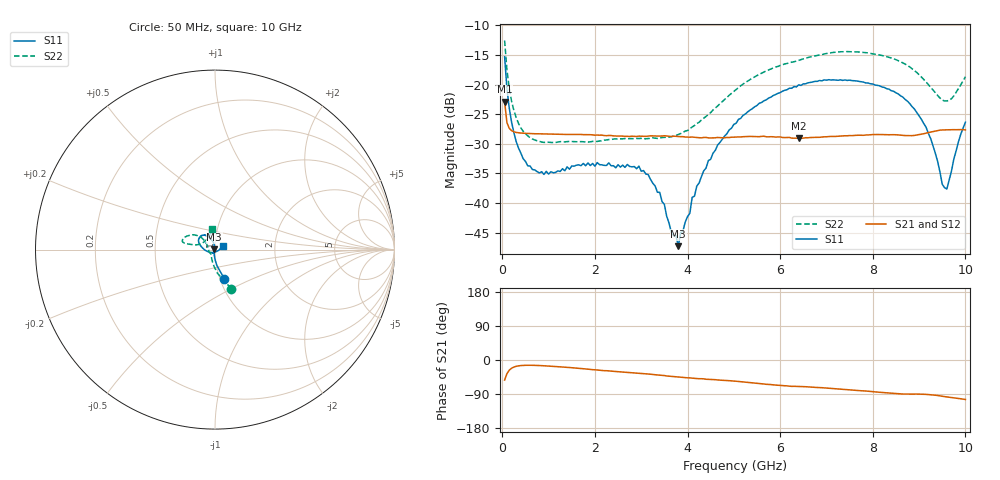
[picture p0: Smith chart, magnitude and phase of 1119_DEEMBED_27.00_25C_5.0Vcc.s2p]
!Hittite Microwave Corp.
!Digital Attenuator/PhaseShifter Rev 1.4.0
!Filename: C:\DATA\DATA\1119_DEEMBED_27.00_25C_5.0Vcc.s2p
!VNA ID: Agilent Technologies,N5224A,MY51441122,A.10.45.03
!Device type:
!2 Port Calibration.
!Temp(C): 25
!Lot Number:
!Serial Number:
!Operator:
!Misc:
!Attenuator:  27.000
# GHZ S DB R 50.0
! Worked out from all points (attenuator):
!   200 points, 50 MHz to 10 GHz, reference 50 ohm
!   highest |S21| = -22.89 dB at 50 MHz (marker M1); lowest = -29.1 dB at 6.4 GHz (marker M2)
!   lowest |S11| = -47.3 dB at 3.8 GHz (marker M3), VSWR 1.01, Z = 49.6 + j0.0687 ohm
!   |S11| at or under -10 dB: start of sweep to end of sweep
!   |S22| runs from -29.8 to -12.6 dB; largest |S21 - S12| = 0.00013
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0.05  -15.31 -72.2  -22.89 -53.0  -22.90 -53.0  -12.56 -67.4
0.1  -20.72 -82.6  -26.42 -36.2  -26.41 -36.1  -17.51 -83.9
0.2  -26.33 -91.3  -27.78 -21.7  -27.78 -21.7  -22.79 -100.5
0.35  -30.72 -98.1  -28.14 -15.5  -28.15 -15.5  -26.56 -114.7
0.55  -33.72 -106.2  -28.26 -13.8  -28.26 -13.9  -28.66 -126.3
0.9  -35.18 -113.4  -28.34 -15.2  -28.35 -15.2  -29.77 -135.8
1.75  -33.32 -121.9  -28.46 -23.1  -28.46 -23.1  -29.66 -140.7
2.95  -33.78 -113.3  -28.71 -34.8  -28.72 -34.9  -29.12 -160.0
3.4  -38.20 -124.2  -28.69 -39.8  -28.70 -39.9  -29.02 -173.5
3.8  -47.29 170.8  -28.77 -44.9  -28.78 -45.0  -28.45 170.6
4.05  -41.73 115.8  -28.89 -47.2  -28.91 -47.3  -27.48 160.0
4.1  -39.04 112.2  -28.87 -47.9  -28.87 -47.9  -27.17 158.3
4.45  -32.83 99.0  -29.01 -51.2  -29.02 -51.3  -25.05 146.3
5.05  -26.53 105.5  -28.87 -56.1  -28.89 -56.1  -20.83 138.8
6.4  -20.05 125.2  -29.08 -69.9  -29.10 -69.9  -15.93 149.9
6.7  -19.57 130.8  -28.93 -71.7  -28.94 -71.7  -15.25 153.9
8.35  -20.78 160.7  -28.48 -87.1  -28.48 -87.1  -15.41 168.1
8.75  -22.82 171.3  -28.62 -89.8  -28.62 -89.9  -16.78 168.1
9.15  -27.18 -165.4  -28.21 -90.7  -28.22 -90.7  -19.56 165.4
9.5  -36.83 -107.6  -27.67 -95.7  -27.69 -95.7  -22.62 143.9
9.6  -37.64 -57.0  -27.65 -97.4  -27.67 -97.4  -22.78 132.3
10  -26.37 28.1  -27.66 -104.2  -27.66 -104.2  -18.68 98.5
